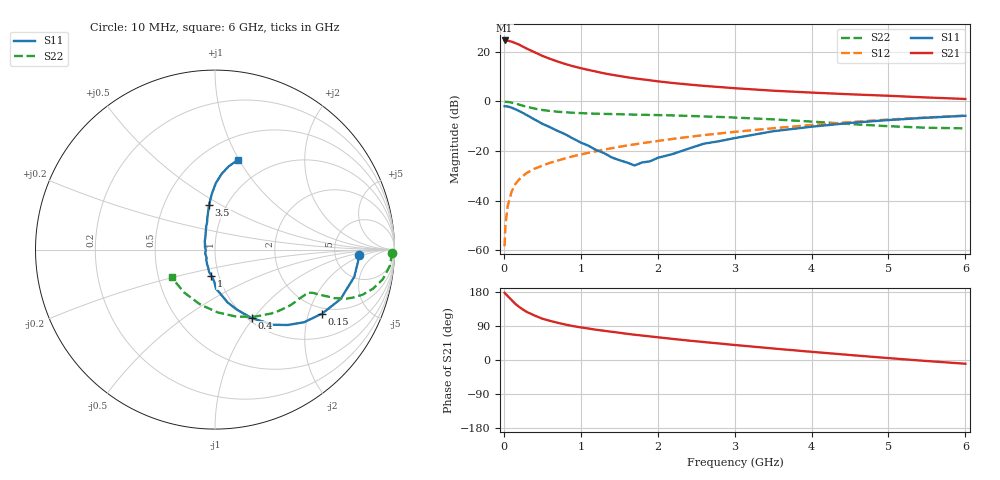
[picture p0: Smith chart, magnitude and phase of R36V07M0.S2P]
! SIEMENS Small Signal Semiconductors
! BFR181
! Si NPN RF Bipolar Junction Transistor in SOT23
! VCE = 6 V  IC = 7 mA
! Common Emitter S-Parameters:  May  1996
# GHz  S  MA  R  50
!  f  S11  S21  S12  S22
! GHz  MAG  ANG  MAG  ANG  MAG  ANG  MAG  ANG
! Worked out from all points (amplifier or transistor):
!   36 points, 10 MHz to 6 GHz, reference 50 ohm
!   highest |S21| = 24.6 dB at 10 MHz (marker M1)
!   |S21| within 3 dB of that: start of sweep to 280 MHz
!   unconditionally stable (mu >= 1): 994.3 MHz to 2.892 GHz
!   at 250 MHz: K = 0.50, MSG = 26.1 dB, |S12| = -30.0 dB
!   at 1.4 GHz: K = 1.05, MAG = 13.5 dB, |S12| = -18.9 dB
!   at 6 GHz: K = 0.86, MSG = 3.4 dB, |S12| = -5.7 dB
!   S11 on the Smith chart (normalised r, x): 10 MHz: 8.86, -1.53; 150 MHz: 1.79, -2.47; 400 MHz: 1.04, -0.98; 1 GHz: 0.92, -0.28; 3.5 GHz: 0.83, +0.44; 6 GHz: 0.73, +0.98
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0.01  0.8026 -2.2  17.04 177.2  0.0012 93.9  0.989 -1.0
0.02  0.8003 -4.5  16.76 174.8  0.0032 81.8  0.9844 -2.1
0.05  0.7905 -11.1  16.82 168.7  0.0077 84.0  0.9791 -5.2
0.1  0.752 -21.5  16.14 158.4  0.0151 79.4  0.9497 -10.0
0.15  0.6956 -30.8  15.04 148.1  0.0216 75.2  0.9067 -13.9
0.2  0.6404 -39.2  14 140.0  0.0268 71.9  0.8614 -16.9
0.25  0.584 -46.0  12.73 132.8  0.0316 69.4  0.8182 -19.0
0.3  0.5292 -52.3  11.63 126.8  0.0362 68.3  0.781 -20.5
0.4  0.4321 -61.9  9.846 117.3  0.044 66.6  0.7188 -22.1
0.5  0.3548 -70.1  8.337 109.0  0.0505 66.1  0.6728 -22.7
0.6  0.3027 -76.6  7.25 103.3  0.0578 66.1  0.6428 -23.2
0.7  0.2542 -82.1  6.398 98.2  0.064 66.4  0.621 -23.5
0.8  0.2174 -88.6  5.694 93.6  0.0712 66.1  0.6047 -23.7
1  0.1485 -97.6  4.699 86.1  0.0851 67.0  0.5817 -24.4
1.1  0.1278 -105.1  4.329 83.0  0.092 67.4  0.5734 -25.0
1.3  0.0912 -119.3  3.711 77.2  0.1067 67.1  0.5614 -26.5
1.6  0.0586 -159.8  3.085 69.2  0.129 66.3  0.5482 -29.3
2.2  0.0874 127.8  2.355 55.6  0.1759 63.8  0.5218 -36.5
3.5  0.2503 97.6  1.65 30.4  0.2879 54.0  0.435 -59.1
4.5  0.3687 89.4  1.396 13.2  0.3832 43.5  0.35 -87.6
5.5  0.4706 80.6  1.203 -2.7  0.4754 31.2  0.2945 -125.8
6  0.5139 75.8  1.123 -9.9  0.5186 24.3  0.2868 -147.5
